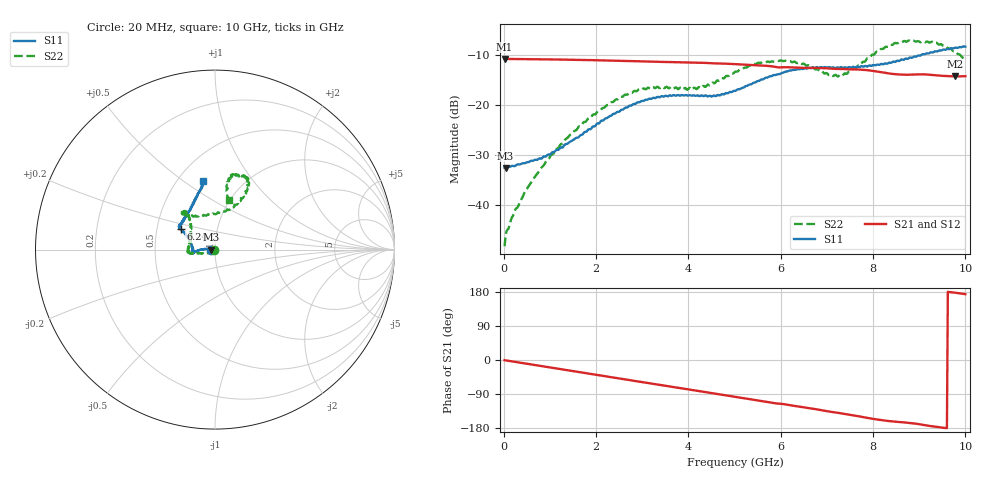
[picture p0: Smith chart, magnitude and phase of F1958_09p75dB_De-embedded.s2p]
! Integrated Device Technology
! Corporate Headquarters
! 6024 Silver Creek Valley Road
! San Jose, CA 95138  USA
! Phone:  1-408-284-8200
! Toll Free:  1-800-223-1366
! Webpage:  http://www.idt.com/
! Timing and RF Division
! 515 Groton Road, Suite 102
! Westford, MA 01886-6024
! Device:  F1958
! Description: 7-bit 0.25 dB Digital Step Attenuator
! Frequency:  0.001 -  6.000 GHz
! Package:  4x4 mm Thin QFN Plastic Package: 24 pin
! Ports:  2 RF, 12 DC
!  Pin  1  = D0
!  Pin  2  = VDD
!  Pin  3  = VMODE
!  Pin  4  = GND
!  Pin  5  = RF1  =  Port 1
!  Pin  6  = GND
!  Pin  7  = GND
!  Pin  8  = GND
!  Pin  9  = GND
!  Pin 10  = GND
!  Pin 11  = GND
!  Pin 12  = GND
!  Pin 13  = GND
!  Pin 14  = RF2  =  Port 2
!  Pin 15  = GND
!  Pin 16  = LE
!  Pin 17  = CLK
!  Pin 18  = DATA
!  Pin 19  = D6
!  Pin 20  = D5
!  Pin 21  = D4
!  Pin 22  = D3
!  Pin 23  = D2
!  Pin 24  = D1
! State:  39
! Atten State:  9.75 dB
! Voltage:  +3.30 Volts
! Current:  0.258 mA
! Data:  The device was measured on a F1958 evaluation board which has
!  individual transmission lines to the RF pins.  Data was collected
!  using a calibrated network analyzer.  The evaluation board was
!  de-embedded using Automatic Fixture Removal (AFR).
!  The reference plane is the edge of the package pin.
! Misc:
!  Action Tracker AT0419
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# GHz S dB R 50
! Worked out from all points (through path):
!   500 points, 20 MHz to 10 GHz, reference 50 ohm
!   highest |S21| = -10.71 dB at 20 MHz (marker M1); lowest = -14.2 dB at 9.78 GHz (marker M2)
!   group delay of S21, straight-line fit = 52.5 ps
!   lowest |S11| = -32.6 dB at 40 MHz (marker M3), VSWR 1.05, Z = 47.7 - j0.0736 ohm
!   |S11| at or under -10 dB: start of sweep to 9.033 GHz
!   |S22| runs from -48.3 to -7.0 dB; largest |S21 - S12| = 0.00078
!   S11 on the Smith chart (normalised r, x): 20 MHz: 0.95, -0.00; 6.24 GHz: 0.66, +0.16; 10 GHz: 0.67, +0.60
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0.02  -32.57 -178.2  -10.71 -0.5  -10.71 -0.5  -48.32 -148.7
0.04  -32.61 -178.1  -10.72 -0.9  -10.72 -0.9  -46.30 -142.8
0.22  -32.26 178.1  -10.75 -4.5  -10.75 -4.5  -41.84 -138.3
0.6  -31.17 174.4  -10.79 -11.9  -10.79 -11.9  -35.46 -139.3
1.14  -29.01 175.4  -10.85 -22.4  -10.84 -22.4  -28.83 -148.2
1.7  -25.95 177.0  -10.94 -33.2  -10.93 -33.2  -23.86 -161.1
2.58  -20.91 -176.8  -11.13 -50.3  -11.11 -50.3  -18.31 -170.4
3.36  -18.41 -171.6  -11.32 -65.3  -11.32 -65.4  -16.52 -174.9
4.22  -18.13 -174.7  -11.50 -81.8  -11.51 -81.9  -16.40 156.9
4.64  -17.96 176.0  -11.64 -89.9  -11.65 -89.9  -15.06 140.9
5.02  -17.13 164.8  -11.76 -97.2  -11.77 -97.3  -13.27 130.7
5.56  -14.97 153.5  -12.05 -107.6  -12.06 -107.6  -11.56 128.0
6.24  -13.01 149.2  -12.43 -120.0  -12.45 -120.0  -11.38 132.2
6.68  -12.49 147.1  -12.54 -128.2  -12.56 -128.1  -12.40 126.9
7.08  -12.48 144.0  -12.66 -136.6  -12.67 -136.5  -13.84 108.5
7.32  -12.40 142.0  -12.75 -141.1  -12.75 -140.9  -14.07 91.5
7.9  -12.13 130.4  -13.01 -153.2  -13.00 -153.2  -10.54 64.6
8.34  -11.50 120.9  -13.63 -161.1  -13.63 -161.2  -8.16 61.8
8.76  -10.68 112.5  -13.90 -165.7  -13.91 -165.7  -7.07 66.2
9.24  -9.44 104.7  -13.92 -174.3  -13.93 -174.3  -7.42 75.3
9.78  -8.47 100.2  -14.24 177.4  -14.27 177.4  -9.19 78.5
10  -8.27 99.7  -14.19 173.6  -14.23 173.7  -10.91 74.4
